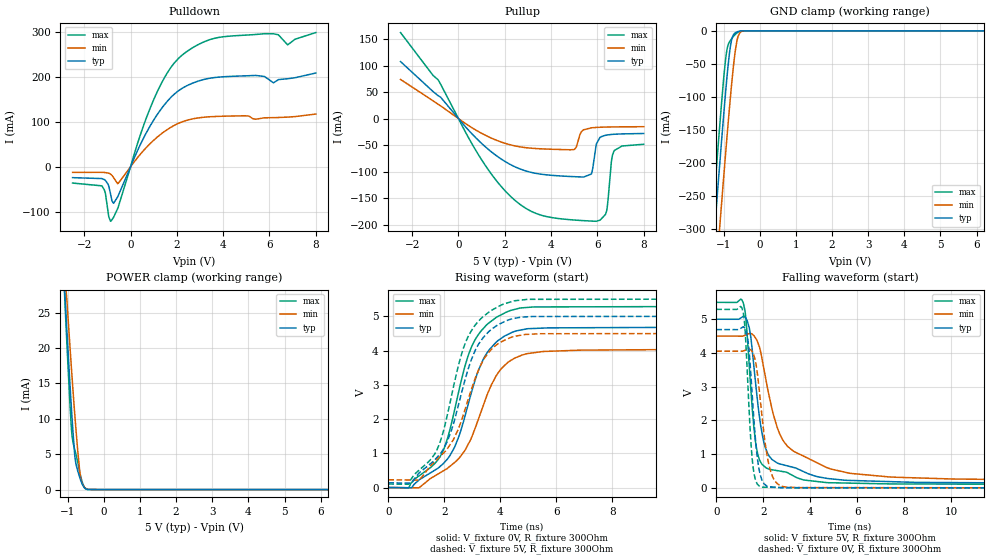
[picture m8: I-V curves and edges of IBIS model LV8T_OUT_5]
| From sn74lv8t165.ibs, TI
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[Model]   LV8T_OUT_5
Model_type   3-state
Polarity   Non-Inverting
Vmeas = 2.5
Vref = 0
Cref = 50pF
Rref = 1000
|   typ   min   max
C_comp   1.25pF   1.25pF   1.25pF
[Voltage Range]   5   4.5   5.5
[Temperature Range]   27   125   -40
[Pullup Reference]   5   4.5   5.5
[Pulldown Reference]   0   0   0
[Power Clamp Reference]   5   4.5   5.5
[GND Clamp Reference]   0   0   0
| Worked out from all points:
|   slope of the pulldown table from 0 to 0.75 V, typ, clamps not added: 9.14 ohm
|   slope of the pullup table from 0 to 0.75 V, typ, clamps not added: 20.6 ohm
|   GND clamp passes 1 mA (typ) near -0.60 V on its own axis
|   POWER clamp passes 1 mA (typ) near -0.62 V on its own axis
|   falling waveform, V_fixture 5V, R_fixture 300Ohm: 20-80 % time 595ps typ, 1.31ns min, 385ps max; typ from 5 V to 0.138 V
|   rising waveform, V_fixture 0V, R_fixture 300Ohm: 20-80 % time 1.19ns typ, 1.37ns min, 1.1ns max; typ from 0 V to 4.69 V
|   rising waveform, V_fixture 5V, R_fixture 300Ohm: 20-80 % time 1.16ns typ, 1.29ns min, 1.08ns max; typ from 0.138 V to 5 V
|   falling waveform, V_fixture 0V, R_fixture 300Ohm: 20-80 % time 308ps typ, 428ps min, 242ps max; typ from 4.69 V to 0 V
[Pulldown]
|   Voltage   I(typ)   I(min)   I(max)
-2.5V     -23.88mA   -12.08mA   -35.89mA
-1.24V    -25.92mA   -12.06mA   -42.08mA
-1.093V   -29.64mA   -12.57mA   -57.01mA
-851.5mV  -62.86mA   -16.45mA   -120.6mA
-736mV    -80.64mA   -23.26mA   -112.3mA
-526mV    -63.41mA   -36.33mA   -88.58mA
870.5mV   93mA       52.88mA    133.4mA
2.12V     171mA      97.9mA     243.5mA
3.789V    199.5mA    112.3mA    287.6mA
6.173V    186.9mA    109.5mA    296mA
6.782V    196mA      110.7mA    271.5mA
8V        208.7mA    117.5mA    298.6mA
[GND Clamp]
|   Voltage   I(typ)   I(min)   I(max)
-2.5V     -1.223A    -1.308A    -1.175A
-1.313V   -348.7mA   -443.1mA   -291.5mA
-1.23V    -288.7mA   -383.5mA   -231.1mA
-1.135V   -222.2mA   -317.2mA   -164.4mA
-1.062V   -171.5mA   -266.3mA   -114.2mA
-977.5mV  -115.5mA   -209.1mA   -61.53mA
-904mV    -69.7mA    -160.4mA   -28.36mA
-778mV    -14.25mA   -82.1mA    -12.14mA
-631mV    -1.745mA   -15.92mA   -3.28mA
-547mV    -376.1uA   -2.828mA   -696.1uA
-431.5mV  -13.18uA   -139.1uA   -11.3uA
8V        0A         0A         0A
[Pullup]
|   Voltage   I(typ)   I(min)   I(max)
-2.5V     107.4mA    73.75mA    162.2mA
-872.5mV  42.97mA    26.7mA     72.89mA
1.458V    -64.13mA   -37.67mA   -106.9mA
3.223V    -102.5mA   -56.29mA   -176.7mA
4.997V    -109.7mA   -58.49mA   -191.5mA
5.742V    -104.7mA   -17.58mA   -193.5mA
5.952V    -48.4mA    -16.84mA   -193.9mA
6.11V     -35.84mA   -16.5mA    -191.9mA
6.404V    -31.21mA   -16.1mA    -173.9mA
6.604V    -30.12mA   -15.93mA   -82.23mA
6.719V    -29.73mA   -15.85mA   -61.15mA
8V        -28.29mA   -15.45mA   -48.57mA
[POWER Clamp]
|   Voltage   I(typ)   I(min)   I(max)
-2.5V     127.4mA    101.1mA    159.7mA
-1.145V   33.97mA    32.77mA    34.17mA
-1.04V    24.15mA    27.93mA    22.63mA
-1.03V    23.19mA    27.36mA    21.5mA
-946mV    15.68mA    20.9mA     12.95mA
-893.5mV  11.27mA    16.96mA    8.379mA
-862mV    8.817mA    14.67mA    6.971mA
-799mV    4.62mA     10.32mA    5.548mA
-652mV    1.487mA    1.984mA    2.164mA
-589mV    682.9uA    753.2uA    922.8uA
-494.5mV  92.62uA    157.9uA    70.62uA
8V        0A         0A         0A
[Ramp]
R_load = 300
|   typ   min   max
dV/dt_r   2.81573/1.1946e-09   2.43118/1.36559e-09   3.17529/1.0996e-09
dV/dt_f   2.91711/5.90539e-10   2.56385/1.30589e-09   3.23809/3.84541e-10
[Falling Waveform]
V_fixture = 5V
V_fixture_min = 4.5V
V_fixture_max = 5.5V
R_fixture = 300Ohm
C_fixture = 0F
|   Time   V(typ)   V(min)   V(max)
0s        5V         4.5V       5.5V
1.154ns   5.089V     4.505V     5.472V
1.274ns   5.011V     4.539V     4.913V
1.402ns   4.755V     4.575V     3.63V
1.668ns   3.138V     4.443V     1.377V
1.887ns   1.857V     4.03V      764.5mV
2.119ns   1.134V     3.182V     593.9mV
2.895ns   675.5mV    1.35V      476.1mV
4.871ns   268mV      559.2mV    151.8mV
15ns      138mV      226.6mV    103.1mV
[Rising Waveform]
V_fixture = 0V
V_fixture_min = 0V
V_fixture_max = 0V
R_fixture = 300Ohm
C_fixture = 0F
|   Time   V(typ)   V(min)   V(max)
0s        170.2uV    313.6uV    108.7uV
722.6ps   -6.958mV   -6.132mV   -6.362mV
1.797ns   579.6mV    405.7mV    838.4mV
2.134ns   856.6mV    575.1mV    1.493V
2.519ns   1.49V      851.3mV    2.82V
3.023ns   2.925V     1.563V     4.195V
3.509ns   3.91V      2.662V     4.745V
4.228ns   4.453V     3.621V     5.125V
5.527ns   4.655V     3.971V     5.272V
15ns      4.693V     4.052V     5.292V
[Rising Waveform]
V_fixture = 5V
V_fixture_min = 4.5V
V_fixture_max = 5.5V
R_fixture = 300Ohm
C_fixture = 0F
|   Time   V(typ)   V(min)   V(max)
0s        138mV      226.6mV    103.1mV
722.6ps   130.2mV    220.1mV    96.22mV
1.128ns   445.1mV    242.7mV    528.6mV
1.887ns   1.019V     939.3mV    1.428V
2.246ns   1.652V     1.301V     2.635V
2.792ns   3.292V     2.417V     4.303V
3.372ns   4.359V     3.689V     4.98V
4.01ns    4.789V     4.244V     5.318V
5.389ns   4.993V     4.49V      5.494V
15ns      5V         4.5V       5.5V
[Falling Waveform]
|Gnd
V_fixture = 0V
V_fixture_min = 0V
V_fixture_max = 0V
R_fixture = 300Ohm
C_fixture = 0F
|   Time   V(typ)   V(min)   V(max)
0s        4.693V     4.052V     5.292V
1.133ns   4.77V      4.055V     5.238V
1.236ns   4.693V     4.08V      4.569V
1.354ns   4.337V     4.108V     2.924V
1.53ns    2.75V      4.034V     857mV
1.696ns   1.217V     3.644V     187.6mV
1.864ns   410.4mV    2.665V     32.55mV
2.279ns   30.29mV    577.9mV    16.29mV
2.816ns   5.975mV    42.09mV    9.861mV
15ns      170.3uV    313.7uV    108.8uV
